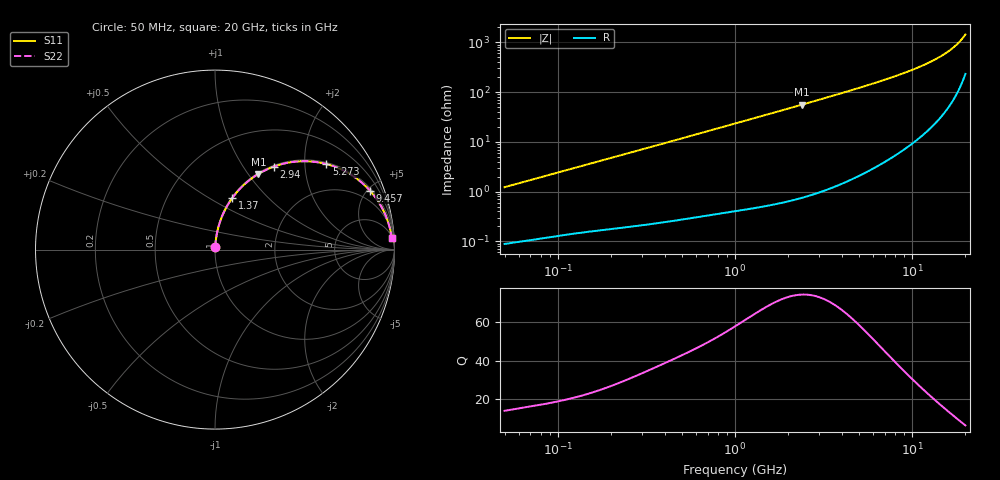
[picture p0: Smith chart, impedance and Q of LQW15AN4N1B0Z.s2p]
!Murata Part Number: LQW15AN4N1B0Z
!These Parameters are Measured in Series Mode Connection
!  o--[Z]--o
!Port1  Port2
!  o-------o
!Freq. Start=50[MHz] Stop=20[GHz], 401[Steps]
# Hz S RI R 50
!Freq.(Hz) S11(Real) S11(Imag) S21(Real) S21(Imag) S12(Real) S12(Imag) S22(Real) S22(Imag)
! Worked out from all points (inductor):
!   401 points, 50 MHz to 20 GHz, reference 50 ohm
!   read as one part in series: L = 3.89 nH near 51.52 MHz
!   highest Q = 74.6 at 2.384 GHz (marker M1), where L = 3.74 nH
!   S11 on the Smith chart (normalised r, x): 50 MHz: 1.00, +0.02; 1.37 GHz: 1.01, +0.64; 2.94 GHz: 1.02, +1.39; 5.273 GHz: 1.05, +2.57; 9.457 GHz: 1.16, +5.18; 20 GHz: 6, +29
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5e7  0.00104 0.0123  0.999 -0.0123  0.999 -0.0123  0.00104 0.0123
1.364002e8  0.00256 0.0325  0.9974 -0.0325  0.9974 -0.0325  0.00256 0.0325
2.33884e8  0.00494 0.0551  0.9951 -0.0551  0.9951 -0.0551  0.00494 0.0551
3.721004e8  0.00992 0.0866  0.9901 -0.0866  0.9901 -0.0866  0.00992 0.0866
6.285508e8  0.0242 0.1434  0.9758 -0.1434  0.9758 -0.1434  0.0242 0.1434
1e9  0.0552 0.22  0.9448 -0.22  0.9448 -0.22  0.0552 0.22
1.369645e9  0.0965 0.2877  0.9035 -0.2877  0.9035 -0.2877  0.0965 0.2877
1.820564e9  0.157 0.3569  0.843 -0.3569  0.843 -0.3569  0.157 0.3569
2.383959e9  0.2414 0.4213  0.7586 -0.4213  0.7586 -0.4213  0.2414 0.4213
2.728004e9  0.2944 0.4491  0.7056 -0.4491  0.7056 -0.4491  0.2944 0.4491
2.940159e9  0.3269 0.4623  0.6731 -0.4623  0.6731 -0.4623  0.3269 0.4623
3.967106e9  0.4731 0.4919  0.5269 -0.4919  0.5269 -0.4919  0.4731 0.4919
5.273168e9  0.6209 0.4764  0.3791 -0.4764  0.3791 -0.4764  0.6209 0.4764
7.442007e9  0.7791 0.4033  0.2209 -0.4033  0.2209 -0.4033  0.7791 0.4033
9.457416e9  0.8628 0.3291  0.1372 -0.3291  0.1372 -0.3291  0.8628 0.3291
1.220001e10  0.9259 0.2411  0.0741 -0.2411  0.0741 -0.2411  0.9259 0.2411
1.482269e10  0.9579 0.172  0.0421 -0.172  0.0421 -0.172  0.9579 0.172
1.597544e10  0.967 0.1455  0.033 -0.1455  0.033 -0.1455  0.967 0.1455
1.721783e10  0.9743 0.1191  0.0257 -0.1191  0.0257 -0.1191  0.9743 0.1191
1.828096e10  0.9791 0.098  0.0209 -0.098  0.0209 -0.098  0.9791 0.098
1.940974e10  0.9829 0.077  0.0171 -0.077  0.0171 -0.077  0.9829 0.077
2e10  0.9845 0.0665  0.0155 -0.0665  0.0155 -0.0665  0.9845 0.0665
